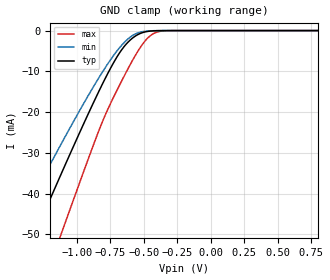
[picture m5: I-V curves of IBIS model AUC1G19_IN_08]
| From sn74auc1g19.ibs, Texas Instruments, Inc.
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[Model]   AUC1G19_IN_08
Model_type  Input
Vinl=0
Vinh=0.8
| variable   typ   min   max
C_comp   2.59pF   2.17pF   2.96pF
[Temperature Range]   40   100   -40
| Ambient temperature   25   85   -40
[Voltage range]   0.8   0.8   0.8
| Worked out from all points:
|   GND clamp passes 1 mA (typ) near -0.55 V on its own axis
[GND Clamp]
| AUC1G19_IN_08
|   Voltage   I(typ)   I(min)   I(max)
-3.6V     -226mA     -190mA     -273.7mA
-1.465V   -61.33mA   -49.31mA   -81.57mA
-1.33V    -51.06mA   -40.82mA   -69.24mA
-1.285V   -47.65mA   -38.02mA   -65.13mA
-1.125V   -35.66mA   -28.21mA   -50.49mA
-1.09V    -33.06mA   -26.11mA   -47.29mA
-815mV    -13.46mA   -10.44mA   -22.78mA
-700mV    -6.409mA   -4.95mA    -14.59mA
-580mV    -1.725mA   -1.12mA    -7.037mA
-450mV    -123.7uA   -59.16uA   -1.218mA
-315mV    -2.431uA   -1.527uA   -21.16uA
800mV     96.17pA    179.9pA    76.88pA
